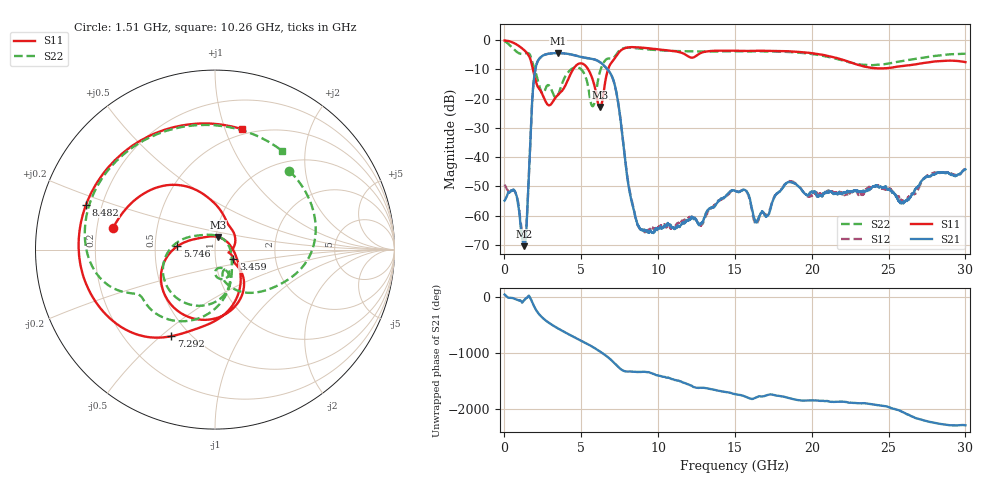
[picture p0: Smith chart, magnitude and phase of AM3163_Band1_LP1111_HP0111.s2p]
!Agilent Technologies,E8364B,MY43040894,A.07.50.67
!Agilent E8364B: A.07.50.67
!Date: Thursday, August 20, 2020 11:58:39
!Correction: S11(Full 2 Port(1,2))
!S21(Full 2 Port(1,2))
!S12(Full 2 Port(1,2))
!S22(Full 2 Port(1,2))
!S2P File: Measurements: S11, S21, S12, S22:
# Hz S  dB  R 50
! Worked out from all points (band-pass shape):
!   3201 points, 10 MHz to 30 GHz, reference 50 ohm
!   highest |S21| = -4.40 dB at 3.487 GHz (marker M1); lowest = -70.5 dB at 1.303 GHz (marker M2)
!   |S21| within 3 dB of the highest: 2.146 GHz to 6.189 GHz (4.043 GHz wide, 97 % of centre)
!   lowest |S11| = -22.8 dB at 6.205 GHz (marker M3), VSWR 1.16, Z = 51.2 + j7.21 ohm
!   |S11| at or under -10 dB: 1.852 GHz to 4.466 GHz (2.614 GHz wide, 82.7 % of centre); 5.454 GHz to 6.743 GHz (1.289 GHz wide, 21.1 % of centre)
!   |S22| runs from -22.6 to -0.4 dB; largest |S21 - S12| = 0.0051
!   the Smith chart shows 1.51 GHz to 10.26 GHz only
!   S11 on the Smith chart (normalised r, x): 1.51 GHz: 0.27, +0.10; 3.459 GHz: 1.22, -0.13; 5.746 GHz: 0.65, +0.02; 7.292 GHz: 0.40, -0.54; 8.482 GHz: 0.14, +0.17; 10.26 GHz: 0.45, +1.14
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1e7  -0.08 -8.0  -54.88 48.5  -49.34 55.1  -0.36 -14.8
7.5975e8  -1.36 -89.1  -52.80 -38.9  -52.91 -38.3  -3.80 -152.0
1.303319e9  -3.48 -158.9  -70.45 -46.1  -69.27 -130.3  -4.58 95.2
1.5095e9  -4.71 168.2  -55.72 1.7  -55.58 47.9  -4.39 46.5
2.043697e9  -14.04 76.4  -9.18 138.6  -9.19 138.5  -11.24 -58.6
2.502919e9  -18.92 14.2  -5.26 -14.6  -5.27 -14.6  -18.20 -63.4
2.905909e9  -22.27 -12.1  -4.59 -101.1  -4.61 -101.1  -15.51 -78.4
3.45885e9  -18.80 -27.0  -4.40 164.2  -4.41 164.2  -19.07 -68.4
3.486966e9  -18.65 -28.2  -4.40 159.8  -4.41 159.8  -18.78 -66.3
4.396038e9  -10.63 -59.2  -4.93 23.8  -4.96 24.0  -9.75 -105.9
5.014581e9  -7.91 -117.4  -5.77 -63.5  -5.75 -63.3  -10.09 -158.1
5.745588e9  -13.52 175.0  -6.44 -172.2  -6.42 -172.3  -22.57 50.2
6.204809e9  -22.85 76.3  -7.45 108.4  -7.48 108.2  -10.95 -81.0
7.291947e9  -5.33 -116.8  -18.07 -139.9  -18.04 -139.2  -4.80 -156.3
8.482175e9  -2.38 160.8  -59.49 103.3  -59.55 103.2  -2.70 131.0
1.000979e10  -3.11 88.3  -64.45 34.6  -64.04 35.4  -3.45 65.6
1.026283e10  -3.25 77.5  -64.32 15.7  -63.21 21.6  -3.54 55.9
1.5005e10  -3.59 -71.9  -51.51 60.3  -51.26 60.8  -3.79 -92.5
2.000958e10  -4.43 162.8  -51.90 -51.2  -53.32 -49.0  -4.71 135.4
2.274617e10  -7.99 59.7  -51.59 -95.9  -52.09 -101.3  -7.93 20.4
2.500479e10  -9.50 -62.9  -50.94 -171.7  -50.85 -175.2  -7.97 -93.2
3e10  -7.48 104.7  -44.19 -137.6  -43.75 -134.6  -4.62 100.4
